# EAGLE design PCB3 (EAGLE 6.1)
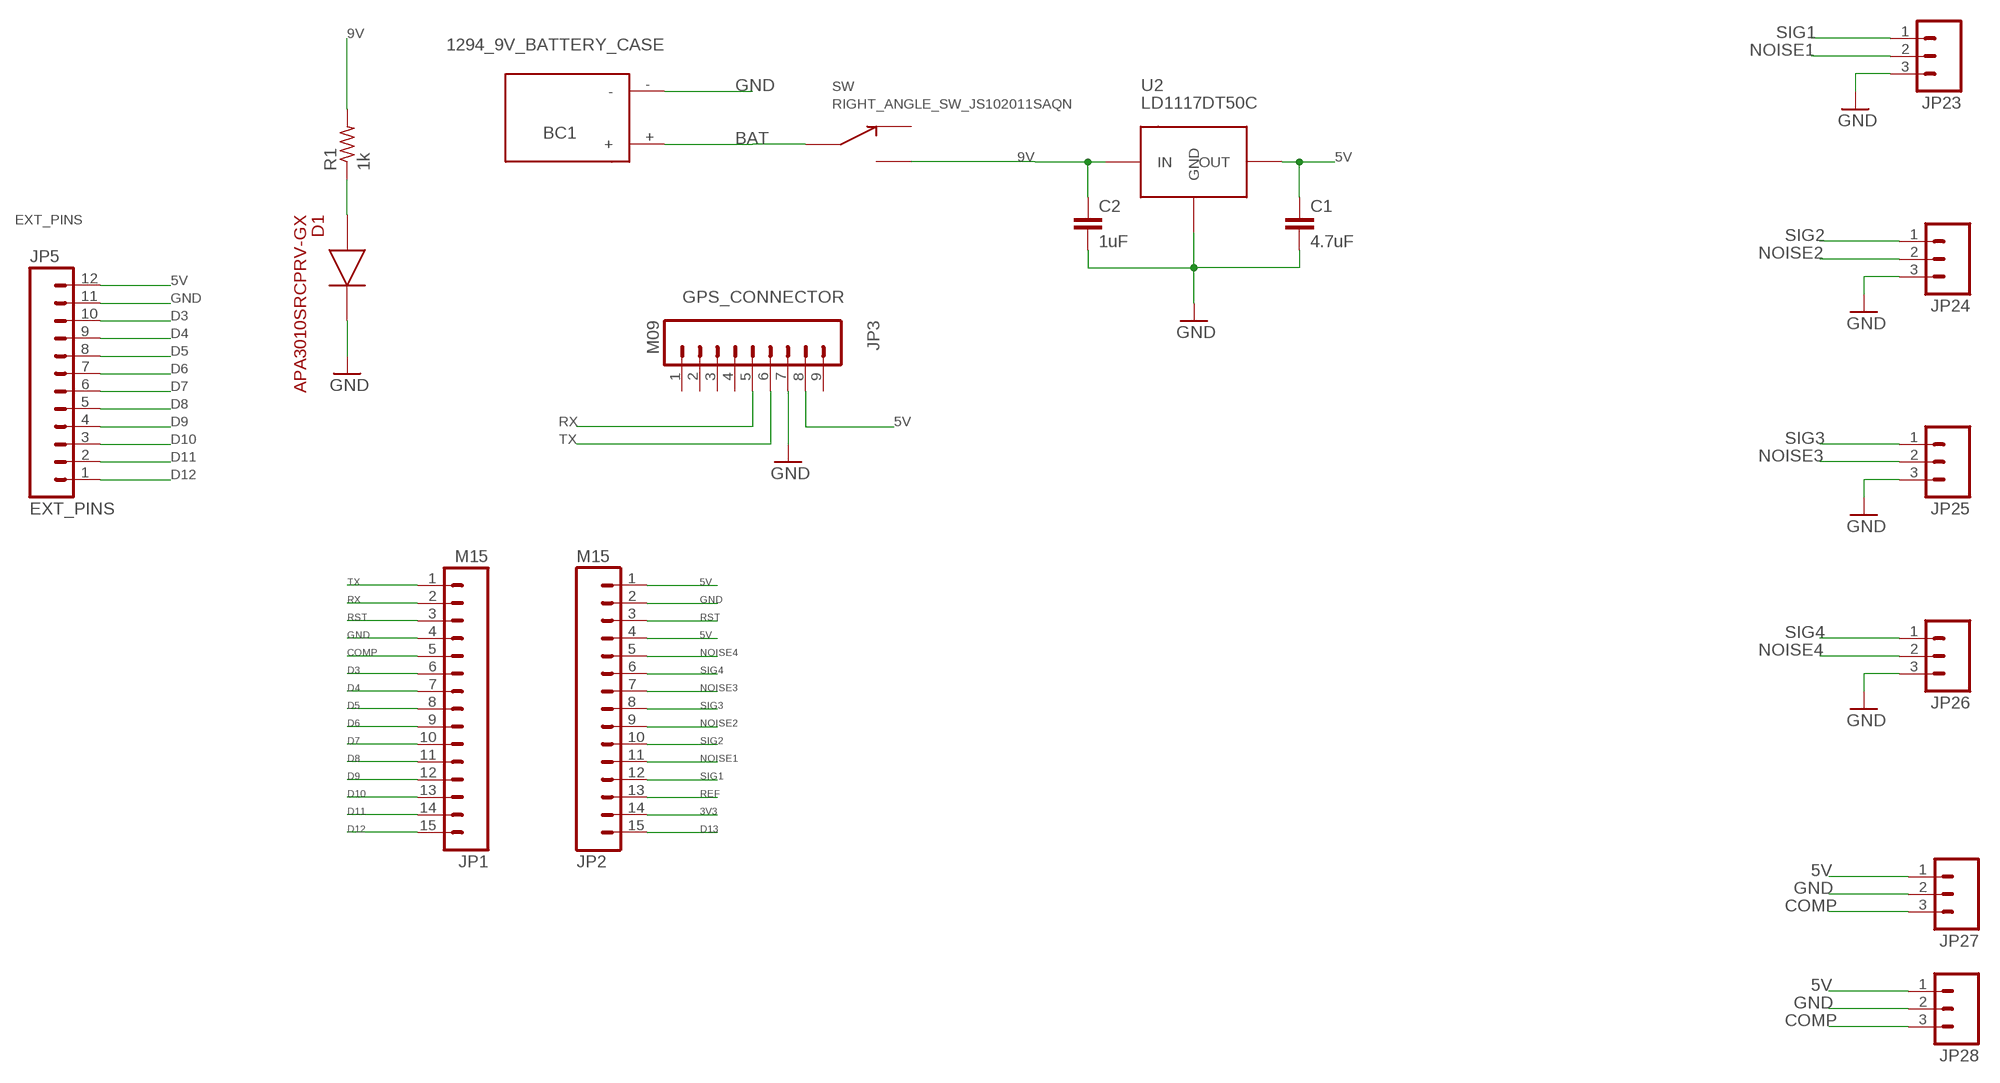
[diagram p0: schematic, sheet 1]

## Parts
BC1  1294_9V_BATTERY_CASE  [1294_BATTERY_CASE]
C1  4.7uF  CAP0805  [0805]
C2  1uF  CAP0603-CAP  [0603-CAP]
D1  APA3010SRCPRV-GX  APA3010SF4C  [APA3010SF4C]
JP1  M15  [1X15]
JP2  M15  [1X15]
JP3  M09  [1X09]
JP5  EXT_PINS  M12PTH  [1X12]
JP23  M03PTH  [1X03]
JP24  M03PTH  [1X03]
JP25  M03PTH  [1X03]
JP26  M03PTH  [1X03]
JP27  M03PTH  [1X03]
JP28  M03PTH  [1X03]
R1  1k  R-US_R1206  [R1206]
SW  RIGHT_ANGLE_SW_JS102011SAQN  [JS102011SAQN]
U2  LD1117DT50C  [DPACK]

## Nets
3V3: JP2.14
5V: C1.1 JP2.1 JP2.4 JP3.8 JP5.12 JP27.1 JP28.1 U2.4(OUT)
9V: C2.1 R1.2 SW.3 U2.3(IN)
BAT: BC1.+ SW.2
COMP: JP1.5 JP27.3 JP28.3
D3: JP1.6 JP5.10
D4: JP1.7 JP5.9
D5: JP1.8 JP5.8
D6: JP1.9 JP5.7
D7: JP1.10 JP5.6
D8: JP1.11 JP5.5
D9: JP1.12 JP5.4
D10: JP1.13 JP5.3
D11: JP1.14 JP5.2
D12: JP1.15 JP5.1
D13: JP2.15
GND: BC1.- C1.2 C2.2 D1.2 JP1.4 JP2.2 JP3.7 JP5.11 JP23.3 JP24.3 JP25.3 JP26.3 JP27.2 JP28.2 U2.1(GND)
N$3: D1.1 R1.1
NOISE1: JP2.11 JP23.2
NOISE2: JP2.9 JP24.2
NOISE3: JP2.7 JP25.2
NOISE4: JP2.5 JP26.2
REF: JP2.13
RST: JP1.3 JP2.3
RX: JP1.2 JP3.5
SIG1: JP2.12 JP23.1
SIG2: JP2.10 JP24.1
SIG3: JP2.8 JP25.1
SIG4: JP2.6 JP26.1
TX: JP1.1 JP3.6
Unconnected: JP3.1 JP3.2 JP3.3 JP3.4 JP3.9 SW.1

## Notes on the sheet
- EXT_PINS
- GPS_CONNECTOR

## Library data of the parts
BC1 = 9V_BATTERY_CASE:1294_9V_BATTERY_CASE
C1 C2 = SparkFun-Capacitors:CAP: Capacitor
D1 = SparkFun-LED:APA3010SF4C: DIO-10854; PROD_ID: DIO-10854
JP1 JP2 = SparkFun-Connectors:M15: Header 15 Standard 15-pin 0.1" header. Use with straight break away headers (SKU : PRT-00116), right angle break away headers (PRT-00553), swiss pins (PRT-00743), machine pins (PRT-00117), and female headers (PRT-00115).
JP3 = SparkFun-Connectors:M09: Header 9 Standard 9-pin 0.1" header. Use with straight break away headers (SKU : PRT-00116), right angle break away headers (PRT-00553), swiss pins (PRT-00743), machine pins (PRT-00117), and female headers (PRT-00115).
JP5 = SparkFun-Connectors:M12: Header 12 Standard 12-pin 0.1" header. Use with straight break away headers (SKU : PRT-00116), right angle break away headers (PRT-00553), swiss pins (PRT-00743), machine pins (PRT-00117), and female headers (PRT-00115).
JP23-JP28 = SparkFun-Connectors:M03: Header 3 Standard 3-pin 0.1" header. Use with straight break away headers (SKU : PRT-00116), right angle break away headers (PRT-00553), swiss pins (PRT-00743), machine pins (PRT-00117), and female headers (PRT-00115). Molex polarized connector foot print use with SKU : PRT-08232 with associated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
R1 = resistor:R-US_: RESISTOR, American symbol
SW = SWITCH_JS102011SAQN:RIGHT_ANGLE_SW_JS102011SAQN
U2 = LD1117DT50C:LD1117DT50C

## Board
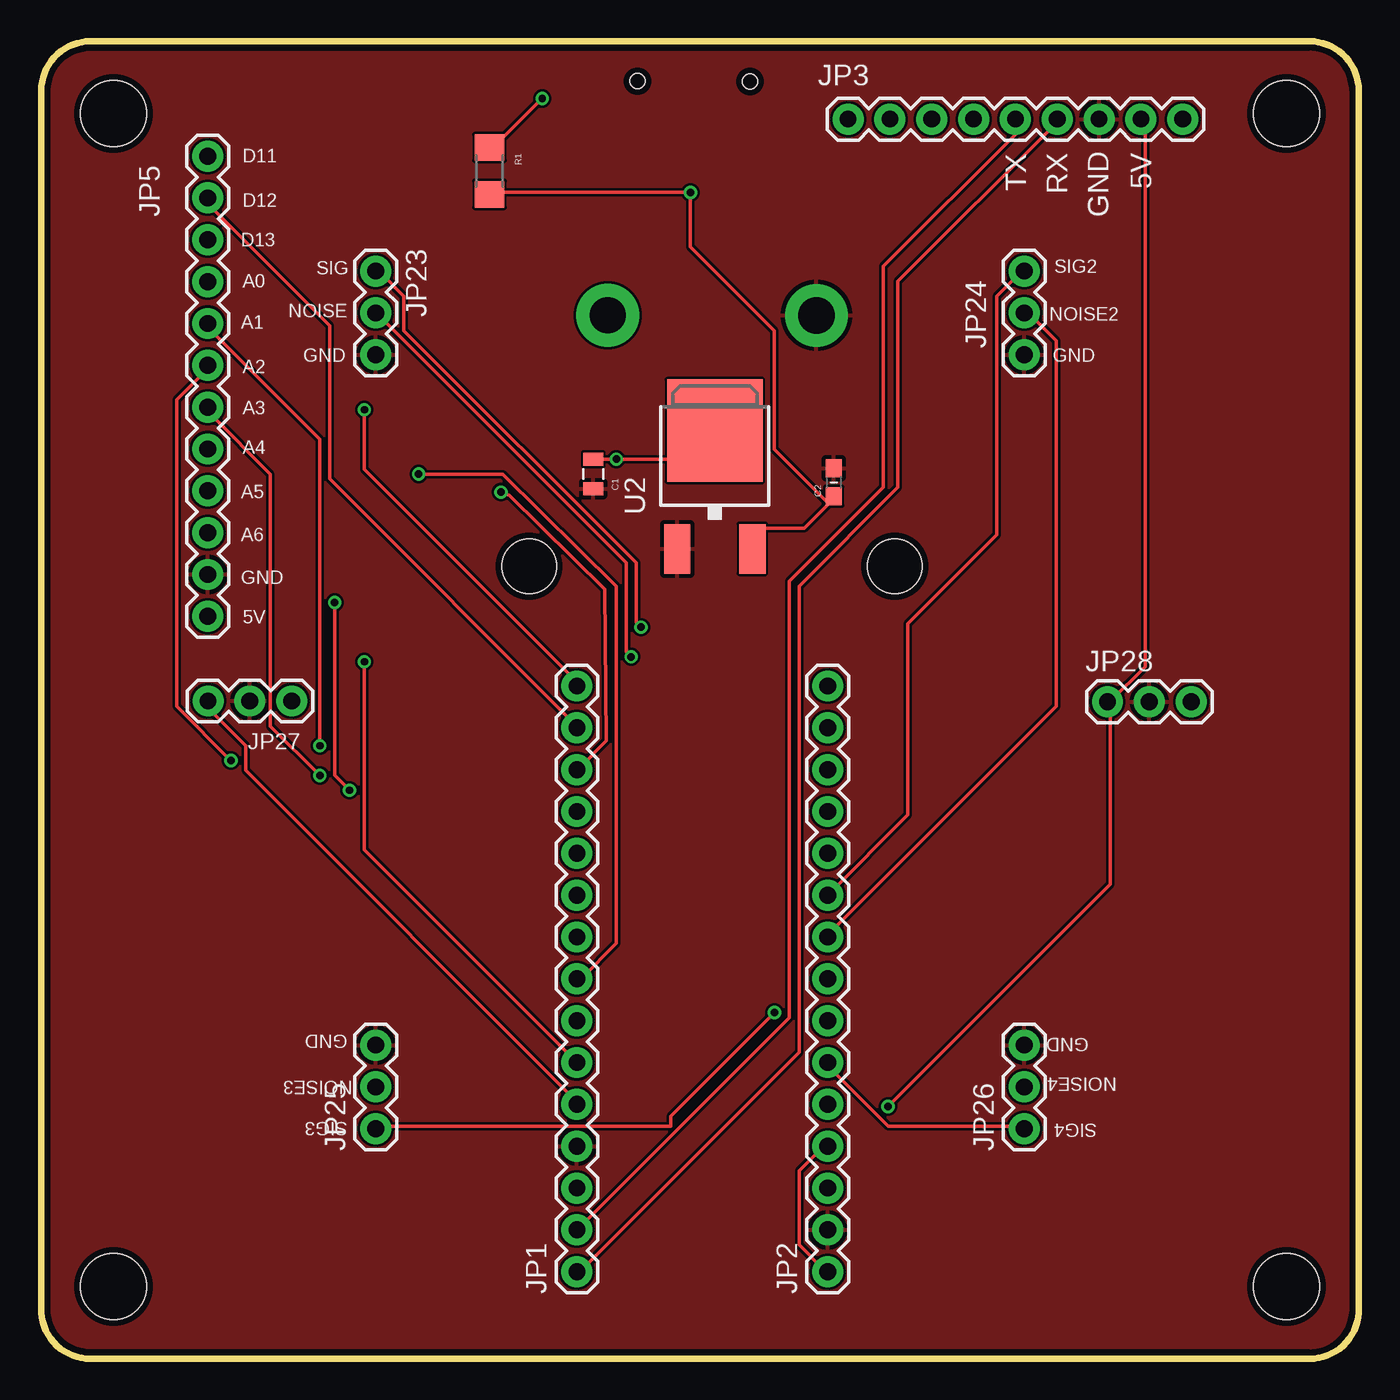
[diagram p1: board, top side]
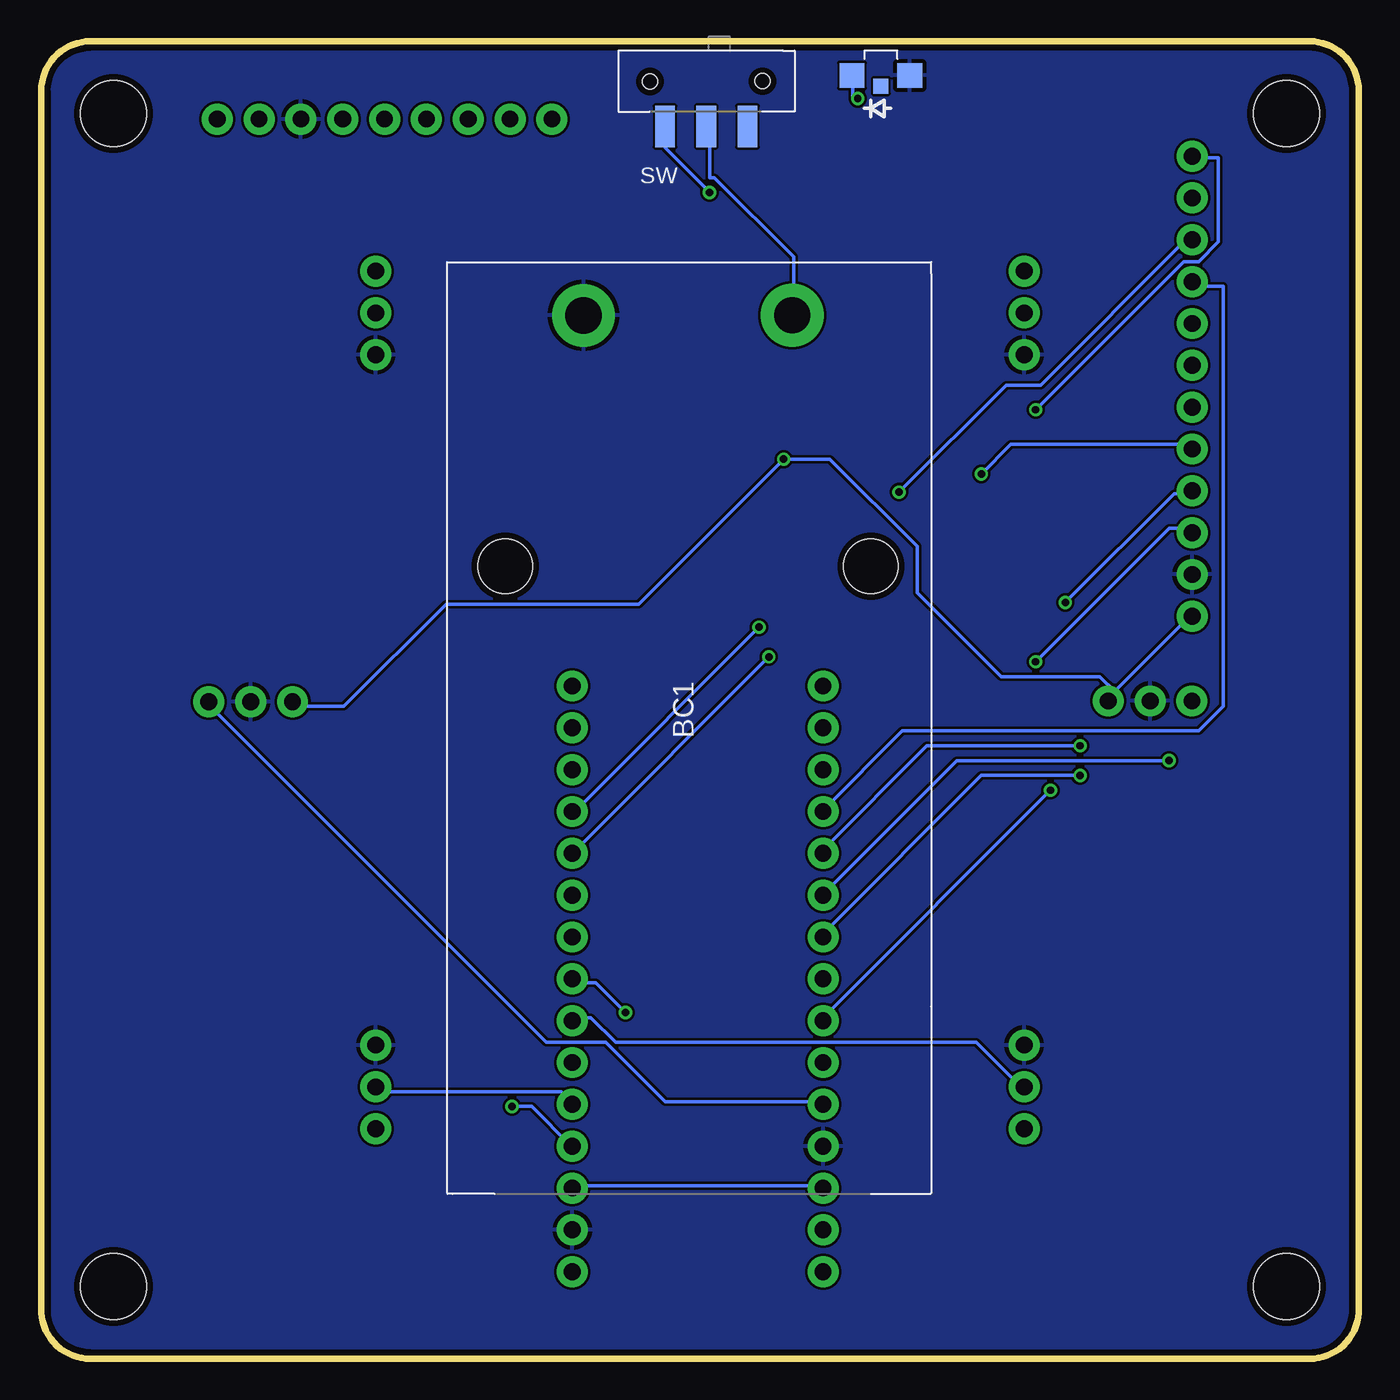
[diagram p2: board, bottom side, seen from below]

Size 80 x 80 mm. Coordinates in mm from the lower left corner, seen from the top.
Outline: 3,0 77,0
Outline: 77,0 3,0
Outline: 3,0 arc-86 0,2.8 0,77 arc-90 3,80 77,80 arc-90 80,77 80,2.8 arc-86 77,0
Copper layers (1*16): Top 0.0356mm / dielectric 1.5011mm / Bottom 0.0356mm
Design rules: minimum track width 6mil, minimum drill 13mil, track to track 6mil, track to pad 6mil, pad to pad 6mil, via to via 6mil, smd to smd 6mil, copper to edge 15mil, drill to drill 6mil, minimum pad ring 7mil, minimum via ring 7mil, stop-mask expansion 3mil, vias tented up to drill 0mil, thermal gap 10mil
Holes 4 mm at 75.6,4.4 4.4,4.4 4.4,75.6 75.6,75.6

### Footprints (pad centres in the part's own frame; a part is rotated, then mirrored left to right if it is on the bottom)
1294_BATTERY_CASE = drill 2.2 pad 3.81: + -15.24,-4.78; - -15.23,-17.45 | hole 3.3: 0,0; 0,-22.2
0805 = smd 0.8 x 1.2: 1 -0.9,0; 2 0.9,0
0603-CAP = smd 1.1 x 1: 1 -0.85,0; 2 0.85,0
APA3010SF4C = smd 1.5 x 1.5: 1 0,-1.75; 2 0,1.75 | smd 0.9 x 0.9: 3 0.65,0
1X15 = drill 1.016 pad 1.88: 1 0,0; 2 2.54,0; 3 5.08,0; 4 7.62,0; 5 10.16,0; 6 12.7,0; 7 15.24,0; 8 17.78,0; 9 20.32,0; 10 22.86,0; 11 25.4,0; 12 27.94,0; 13 30.48,0; 14 33.02,0; 15 35.56,0
1X09 = drill 1.016 pad 1.88: 1 0,0; 2 2.54,0; 3 5.08,0; 4 7.62,0; 5 10.16,0; 6 12.7,0; 7 15.24,0; 8 17.78,0; 9 20.32,0
1X12 = drill 1.016 pad 1.88: 1 0,0; 2 2.54,0; 3 5.08,0; 4 7.62,0; 5 10.16,0; 6 12.7,0; 7 15.24,0; 8 17.78,0; 9 20.32,0; 10 22.86,0; 11 25.4,0; 12 27.94,0
1X03 = drill 1.016 pad 1.88: 1 0,0; 2 2.54,0; 3 5.08,0
R1206 = smd 1.6 x 1.803: 1 -1.422,0; 2 1.422,0
JS102011SAQN = smd 1.2 x 2.5: 1 -2.5,0; 2 0,0; 3 2.5,0 | hole 0.9: 3.41,-2.73; -3.41,-2.75
DPACK = smd 1.6 x 3: 1 -2.28,-4.8; 3 2.28,-4.8 | smd 5.8 x 6.2: 4 0,2.38

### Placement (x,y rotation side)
BC1  29.62,48.12 270 bottom
C1  33.52,53.72 270 top
C2  48.12,53.22 90 top
D1  29.02,77.92 270 bottom
JP1  32.53,5.29 90 top
JP2  47.75,5.29 90 top
JP3  48.99,75.27 0 top
JP5  10.12,73.02 270 top
JP23  20.32,66.04 270 top
JP24  59.69,66.04 270 top
JP25  20.32,13.97 90 top
JP26  59.69,13.97 90 top
JP27  15.21,39.94 180 top
JP28  64.74,39.89 0 top
R1  27.22,72.12 270 top
SW  39.62,74.82 180 bottom
U2  40.9,53.98 0 top

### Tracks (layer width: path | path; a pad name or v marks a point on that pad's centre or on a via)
5V  (via drill 0.45)
  Top 0.2: C1.1 33.72,54.62 v34.92,54.62 40.62,54.62 40.62,56.12 U2.4 | JP2.1 47.52,5.42 46.02,6.92 46.02,11.42 47.52,12.92 JP2.4 | JP3.8 67.02,75.02 67.02,42.02 64.92,39.92 JP28.1 64.92,39.62 64.92,28.82 v51.42,15.32
  Bottom 0.2: 14.82,40.52 10.32,45.02 JP5.12 | 14.82,40.52 15.12,40.22 JP27.1 14.82,40.52 | 14.82,40.52 15.72,41.42 21.72,41.42 26.82,46.52 26.82,49.32 32.12,54.62 v34.92,54.62 43.72,45.82 55.42,45.82 61.62,39.62 64.62,39.62 JP28.1 | v51.42,15.32 50.22,15.32 47.82,12.92 JP2.4
9V  (via drill 0.45)
  Top 0.2: 47.82,51.92 46.32,50.42 43.32,50.42 43.32,49.22 U2.3 | 47.82,51.92 48.12,52.22 C2.1 47.82,51.92 | R1.2 27.42,70.82 v39.42,70.82 39.42,67.52 44.52,62.42 44.52,55.22 47.82,51.92
  Bottom 0.2: v39.42,70.82 42.12,73.52 42.12,74.72 SW.3
BAT
  Bottom 0.2: SW.2 39.42,74.72 39.42,71.72 39.12,71.72 34.32,66.92 34.32,63.62 BC1.+
COMP
  Top 0.2: JP1.5 32.52,15.62 12.42,35.72 12.42,37.22 10.32,39.32 10.32,39.92 JP27.3
  Bottom 0.2: JP28.3 69.72,39.62 49.32,19.22 45.72,19.22 42.12,15.62 32.82,15.62 JP1.5
D3  (via drill 0.45)
  Top 0.2: v19.62,42.32 19.62,30.92 32.52,18.02 JP1.6
  Bottom 0.2: v19.62,42.32 11.52,50.42 10.32,50.42 JP5.10
D4  (via drill 0.45)
  Top 0.2: v18.72,34.52 17.82,35.42 v17.82,45.92
  Bottom 0.2: v18.72,34.52 32.52,20.72 JP1.7 | v17.82,45.92 11.22,52.52 10.32,52.52 JP5.9
D5  (via drill 0.45)
  Top 0.2: v22.92,53.72 28.02,53.72 34.92,46.92 34.92,44.22 34.92,44.12 34.92,25.22 32.82,23.12 JP1.8
  Bottom 0.2: v22.92,53.72 21.12,55.52 10.32,55.52 JP5.8
D6  (via drill 0.45)
  Top 0.2: v16.92,35.42 13.92,38.42 13.92,53.72 10.32,57.32 10.32,57.62 JP5.7
  Bottom 0.2: v16.92,35.42 22.92,35.42 32.52,25.82 JP1.9
D7  (via drill 0.45)
  Top 0.2: v11.52,36.32 8.22,39.62 8.22,58.22 10.02,60.02 10.02,60.32 JP5.6
  Bottom 0.2: v11.52,36.32 24.42,36.32 32.52,28.22 JP1.10
D8  (via drill 0.45)
  Top 0.2: v16.92,37.22 16.92,55.82 10.32,62.42 10.32,62.72 JP5.5
  Bottom 0.2: v16.92,37.22 26.22,37.22 32.52,30.92 JP1.11
D9
  Bottom 0.2: JP1.12 32.52,33.32 27.72,38.12 9.72,38.12 8.22,39.62 8.22,65.12 10.02,65.12 JP5.4
D10  (via drill 0.45)
  Top 0.2: v27.92,52.62 28.42,52.42 34.22,46.72 34.32,37.52 32.82,36.02 JP1.13
  Bottom 0.2: v27.92,52.62 21.42,59.12 19.32,59.12 10.62,67.82 10.32,67.82 JP5.3
D11
  Top 0.2: JP1.14 32.52,38.42 17.52,53.42 17.52,62.72 10.32,69.92 10.32,70.22 JP5.2
D12  (via drill 0.45)
  Top 0.2: v19.62,57.62 19.62,54.02 32.52,41.12 JP1.15
  Bottom 0.2: v19.62,57.62 10.62,66.62 9.72,66.62 8.52,67.82 8.52,72.92 10.02,72.92 JP5.1
GND
  pour Bottom: 3.32,80.02 77.02,80.02 arc-90 80.02,77.02 80.02,3.02 arc-90 77.02,0.02 3.02,0.02 arc-90 0.02,3.02 0.02,76.72 arc-90
  pour Top: 3.32,80.02 77.02,80.02 arc-90 80.02,77.02 80.02,3.02 arc-90 77.02,0.02 3.02,0.02 arc-90 0.02,3.02 0.02,76.72 arc-90
N$3  (via drill 0.45)
  Top 0.2: v30.42,76.52 27.42,73.52 R1.1
  Bottom 0.2: v30.42,76.52 30.72,76.52 30.72,77.72 D1.1
NOISE1  (via drill 0.45)
  Top 0.2: v35.82,42.62 35.52,42.92 35.52,48.32 20.52,63.32 JP23.2
  Bottom 0.2: v35.82,42.62 47.52,30.92 JP2.11
NOISE2
  Top 0.2: JP2.9 47.82,25.82 61.62,39.62 61.62,61.82 59.82,63.62 JP24.2
NOISE3
  Bottom 0.2: JP25.2 20.52,16.52 23.22,19.22 45.12,19.22 46.62,20.72 47.52,20.72 JP2.7
NOISE4
  Bottom 0.2: JP2.5 47.82,15.62 48.42,16.22 59.52,16.22 JP26.2
RST
  Bottom 0.2: JP1.3 32.82,10.52 47.52,10.52 JP2.3
RX
  Top 0.2: JP1.2 32.82,8.12 45.42,20.72 45.42,47.22 51.12,52.92 51.12,66.32 59.22,74.42 59.22,75.02 JP3.5
SIG1  (via drill 0.45)
  Top 0.2: v36.42,44.42 36.12,44.72 36.12,48.32 22.02,62.42 22.02,64.52 20.52,66.02 JP23.1
  Bottom 0.2: v36.42,44.42 47.52,33.32 JP2.12
SIG2
  Top 0.2: JP2.10 47.82,28.22 52.62,33.02 52.62,44.62 58.02,50.02 58.02,64.52 59.52,66.02 JP24.1
SIG3  (via drill 0.45)
  Top 0.2: v44.52,21.02 38.22,14.72 38.22,14.12 20.52,14.12 JP25.1
  Bottom 0.2: v44.52,21.02 46.32,22.82 47.52,22.82 JP2.8
SIG4
  Top 0.2: JP2.6 47.82,17.72 51.42,14.12 59.52,14.12 JP26.1
TX
  Top 0.2: JP1.1 32.82,5.42 46.02,18.62 46.02,46.92 52.02,52.92 52.02,65.42 61.62,75.02 JP3.6

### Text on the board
tPlace: D11 | TX | RX | 5V | D12 | GND | D13 | SIG | SIG2 | A0 | A1 | NOISE | NOISE2 | GND | GND | A2 | A3 | A4 | A5 | A6 | GND | 5V | GND | GND | NOISE3 | NOISE4 | SIG3 | SIG4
